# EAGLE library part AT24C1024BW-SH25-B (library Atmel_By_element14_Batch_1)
Two-wire Serial EEPROM
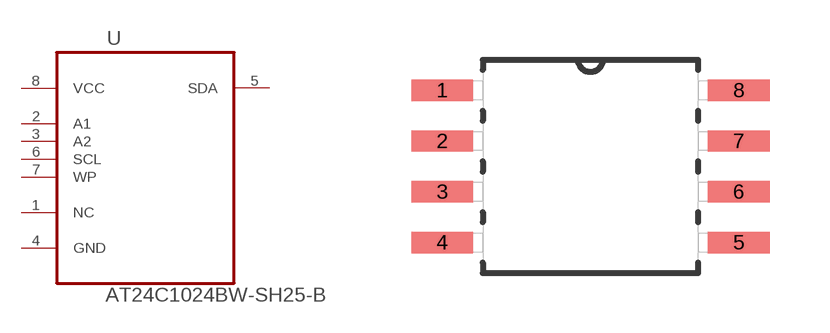
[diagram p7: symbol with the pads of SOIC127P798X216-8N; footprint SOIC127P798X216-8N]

Designator prefix U

## AT24C1024BW-SH25-B (MPN: AT24C1024BW-SH25-B; OC_FARNELL: 1362647; OC_NEWARK: 50M3320; PACKAGE: SOIC-8; SUPPLIER: Atmel)  [SOIC127P798X216-8N]
1  NC  nc
2  A1  in
3  A2  in
4  GND  pas
5  SDA
6  SCL  in
7  WP  in
8  VCC  pwr

## Footprint SOIC127P798X216-8N (pad centres in mm)
smd 1.549 x 0.533: 1 -3.708,1.905; 2 -3.708,0.635; 3 -3.708,-0.635; 4 -3.708,-1.905; 5 3.708,-1.905; 6 3.708,-0.635; 7 3.708,0.635; 8 3.708,1.905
